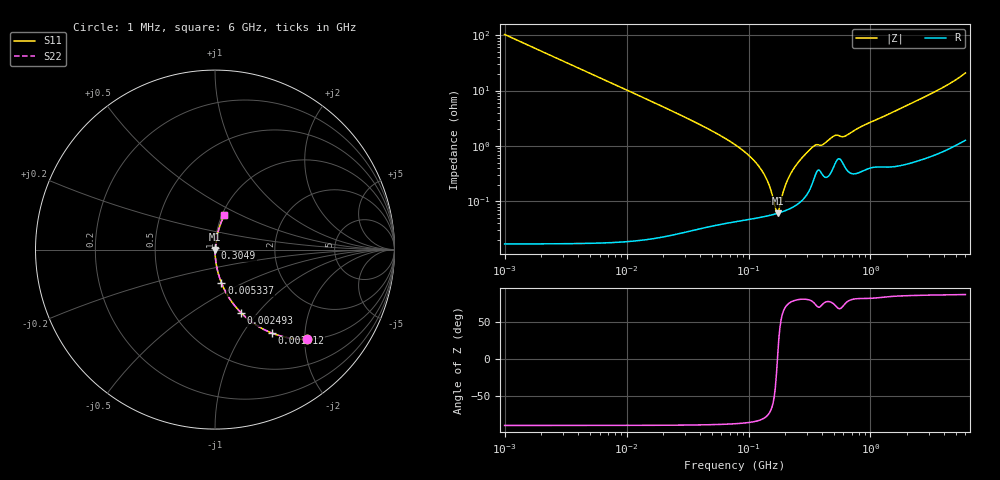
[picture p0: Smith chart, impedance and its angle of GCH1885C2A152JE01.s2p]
!Murata Part Number: GCH1885C2A152JE01
!These Parameters are Measured in Series Mode Connection
!Data Generated on Mar 13, 2026
!  o--ll--o
!Port1  Port2
!  o------o
!Operation Temp=25[degC], DC Bias Voltage=0[V]
!Freq. Start=1000[kHz] Stop=6[GHz] 401[Steps]
# Hz S RI R 50
!Freq.(Hz) S11(Real) S11(Imag) S21(Real) S21(Imag) S12(Real) S12(Imag) S22(Real) S22(Imag)
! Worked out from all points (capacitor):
!   401 points, 1 MHz to 6 GHz, reference 50 ohm
!   read as one part in series: C = 1.55 nF near 1.044 MHz
!   lowest |Z| = 60.9 mohm at 173.2 MHz (marker M1)
!   series resonance near 172.6 MHz, so ESL is about 550 pH
!   S11 on the Smith chart (normalised r, x): 1 MHz: 1.00, -2.06; 1.512 MHz: 1.00, -1.36; 2.493 MHz: 1.00, -0.83; 5.337 MHz: 1.00, -0.39; 304.9 MHz: 1.00, +0.02; 6 GHz: 1.03, +0.42
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1000000  0.5144 -0.4997  0.4856 0.4997  0.4856 0.4997  0.5144 -0.4997
1511688  0.3168 -0.4651  0.6832 0.4651  0.6832 0.4651  0.3168 -0.4651
2492906  0.1457 -0.3526  0.8543 0.3526  0.8543 0.3526  0.1457 -0.3526
4293785  0.0544 -0.2265  0.9456 0.2265  0.9456 0.2265  0.0544 -0.2265
5336962  0.0359 -0.1857  0.9641 0.1857  0.9641 0.1857  0.0359 -0.1857
1.843659e7  0.00325 -0.0549  0.9968 0.0549  0.9968 0.0549  0.00325 -0.0549
7.745967e7  0.000538 -0.0105  0.9995 0.0105  0.9995 0.0105  0.000538 -0.0105
1.027698e8  0.000515 -0.00643  0.9995 0.00643  0.9995 0.00643  0.000515 -0.00643
1.277378e8  0.00053 -0.00364  0.9995 0.00364  0.9995 0.00364  0.00053 -0.00364
1.455431e8  0.000553 -0.00204  0.9994 0.00204  0.9994 0.00204  0.000553 -0.00204
1.658303e8  0.000591 -0.00048  0.9994 0.00048  0.9994 0.00048  0.000591 -0.00048
1.732027e8  0.000607 4.05e-05  0.9994 -4.05e-05  0.9994 -4.05e-05  0.000607 4.05e-05
1.809028e8  0.000626 0.000563  0.9994 -0.000563  0.9994 -0.000563  0.000626 0.000563
2.016844e8  0.000685 0.00189  0.9993 -0.00189  0.9993 -0.00189  0.000685 0.00189
2.200158e8  0.000751 0.00298  0.9992 -0.00298  0.9992 -0.00298  0.000751 0.00298
3.048839e8  0.00144 0.00766  0.9986 -0.00766  0.9986 -0.00766  0.00144 0.00766
3.325952e8  0.00214 0.00914  0.9979 -0.00914  0.9979 -0.00914  0.00214 0.00914
4.045054e8  0.0031 0.01  0.9969 -0.01  0.9969 -0.01  0.0031 0.01
5.138348e8  0.00501 0.0146  0.995 -0.0146  0.995 -0.0146  0.00501 0.0146
6.249308e8  0.00416 0.0145  0.9958 -0.0145  0.9958 -0.0145  0.00416 0.0145
1.428092e9  0.00556 0.0375  0.9944 -0.0375  0.9944 -0.0375  0.00556 0.0375
6e9  0.0523 0.1944  0.9477 -0.1944  0.9477 -0.1944  0.0523 0.1944
